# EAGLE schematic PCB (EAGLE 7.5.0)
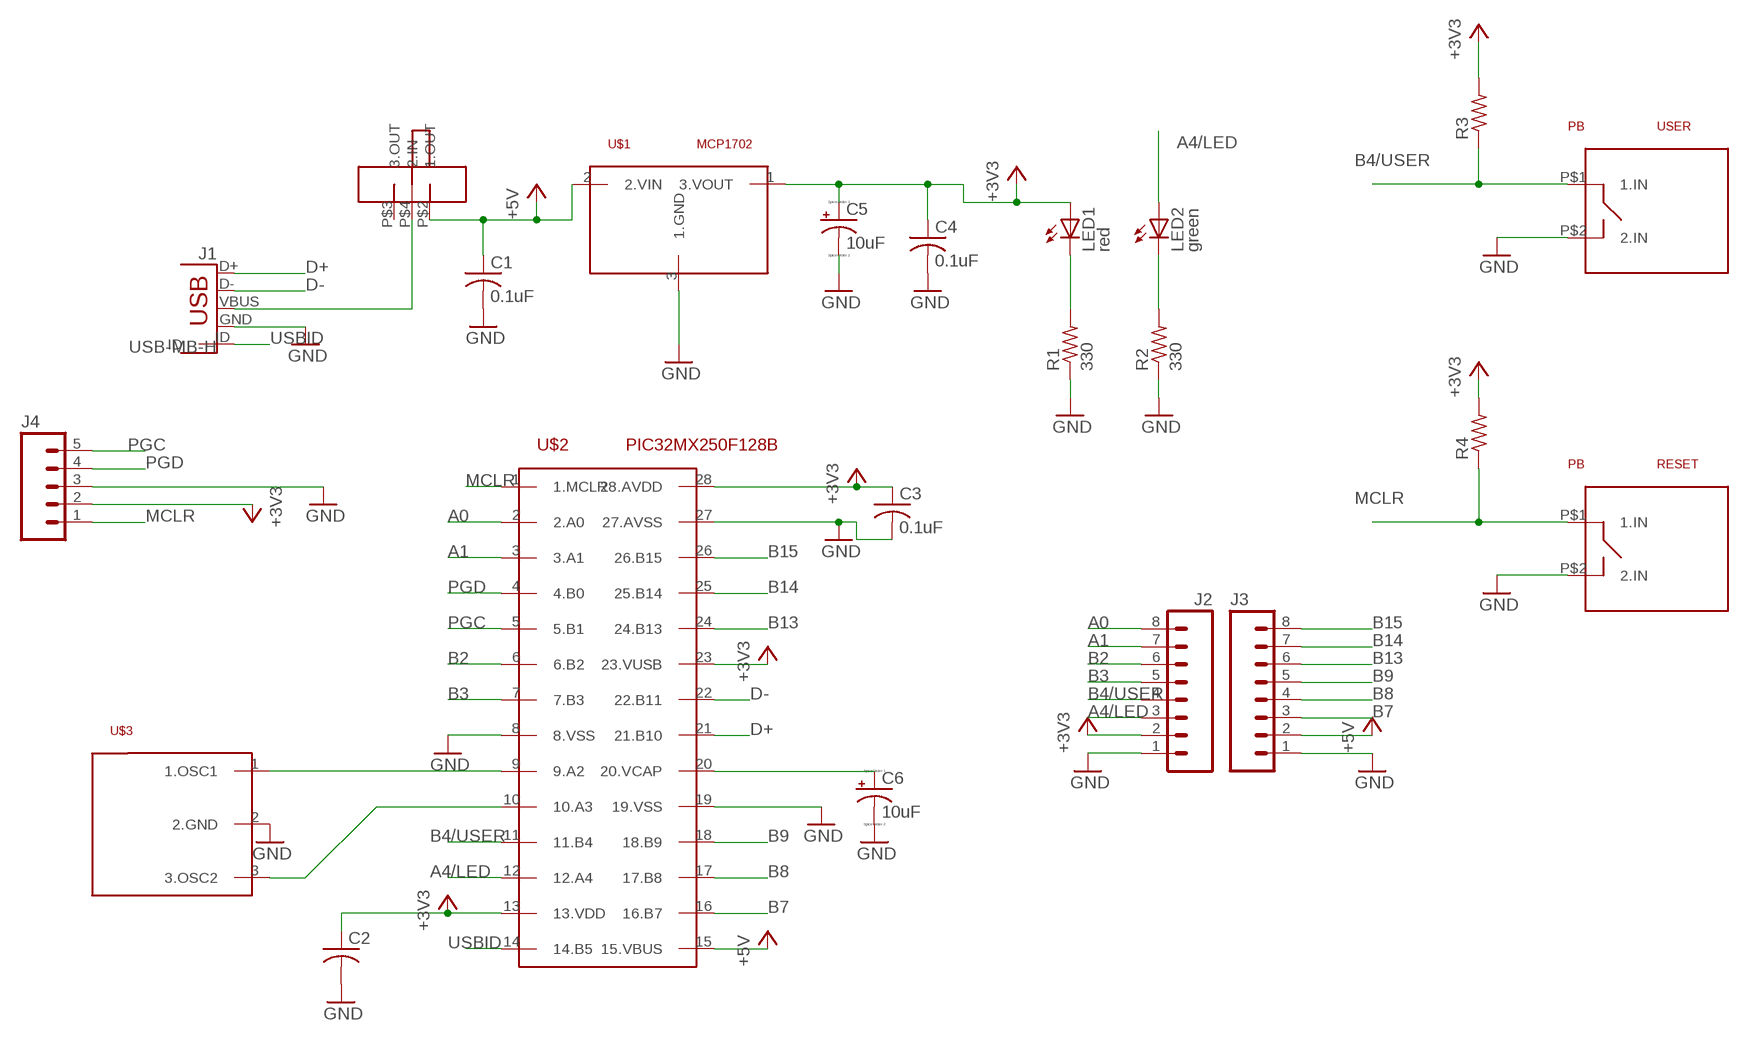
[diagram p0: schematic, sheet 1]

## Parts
C1  0.1uF  C-US025-025X050  [C025-025X050]
C2  C-US025-025X050  [C025-025X050]
C3  0.1uF  C-US025-025X050  [C025-025X050]
C4  0.1uF  C-US025-025X050  [C025-025X050]
C5  10uF  CPOL-USB45181A  [B45181A]
C6  10uF  CPOL-USB45181A  [B45181A]
J1  USB-MB-H  [USB-MB-H]
J2  M08  [1X08_ROUND]
J3  M08  [1X08_ROUND]
J4  M05PTH  [1X05]
LED1  red  LED3MM  [LED3MM]
LED2  green  LED3MM  [LED3MM]
R1  330  R-US_0207/10  [0207/10]
R2  330  R-US_0207/10  [0207/10]
R3  R-US_0207/10  [0207/10]
R4  R-US_0207/10  [0207/10]
RESET  PB  [PUSHBUTTON]
U$1  MCP1702  [TO92]
U$2  PIC32MX250F128B  [DIL28-3]
U$3  CRES  [1X03]
U$4  SLIDE  [SLIDE]
USER  PB  [PUSHBUTTON]

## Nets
+3V3: C2.1 C3.1 C4.1 C5.+ J2.2 J4.2 LED1.A R3.2 R4.2 U$1.1(3.VOUT) U$2.13(13.VDD) U$2.23(23.VUSB) U$2.28(28.AVDD)
+5V: C1.1 J3.2 U$1.2(2.VIN) U$2.15(15.VBUS) U$4.P$2(1.OUT)
A0: J2.8 U$2.2(2.A0)
A1: J2.7 U$2.3(3.A1)
A4/LED: J2.3 LED2.A U$2.12(12.A4)
B2: J2.6 U$2.6(6.B2)
B3: J2.5 U$2.7(7.B3)
B4/USER: J2.4 R3.1 U$2.11(11.B4) USER.P$1(1.IN)
B7: J3.3 U$2.16(16.B7)
B8: J3.4 U$2.17(17.B8)
B9: J3.5 U$2.18(18.B9)
B13: J3.6 U$2.24(24.B13)
B14: J3.7 U$2.25(25.B14)
B15: J3.8 U$2.26(26.B15)
D+: U$2.21(21.B10)
D-: J1.D-
GND: C1.2 C2.2 C3.2 C4.2 C5.- C6.- J1.GND J2.1 J3.1 J4.3 R1.1 R2.1 RESET.P$2(2.IN) U$1.3(1.GND) U$2.8(8.VSS) U$2.19(19.VSS) U$2.27(27.AVSS) U$3.2(2.GND) USER.P$2(2.IN)
MCLR: J4.1 R4.1 RESET.P$1(1.IN) U$2.1(1.MCLR)
N$1: J1.VBUS U$4.P$4(2.IN)
N$2: J1.D+
N$3: U$2.22(22.B11)
N$4: J1.ID
N$5: LED2.K(C) R2.2
N$8: LED1.K(C) R1.2
N$29: C6.+ U$2.20(20.VCAP)
N$36: U$2.10(10.A3) U$3.3(3.OSC2)
N$37: U$2.9(9.A2) U$3.1(1.OSC1)
PGC: J4.5 U$2.5(5.B1)
PGD: J4.4 U$2.4(4.B0)
USBID: U$2.14(14.B5)
Unconnected: U$4.P$3(3.OUT)

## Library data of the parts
C1-C4 = ME 433 PCB lib:C-US: CAPACITOR, American symbol
C5 C6 = ME 433 PCB lib:CPOL-US: POLARIZED CAPACITOR, American symbol
J1 = ME 433 PCB lib:USB: USB Connectors USB-B-PTH is fully proven SKU : PRT-00139/CONN-08278 USB-miniB is fully proven SKU : PRT-00587 USB-A-PCB is untested. USB-A-H is throughly reviewed, but untested. Spark Fun Electronics SKU : PRT-00437 USB-B-SMT is throughly reviewed, but untested. Needs silkscreen touching up.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
J2 J3 = ME 433 PCB lib:M08: Header 8 Standard 8-pin 0.1" header. Use with straight break away headers (SKU : PRT-00116), right angle break away headers (PRT-00553), swiss pins (PRT-00743), machine pins (PRT-00117), and female headers (PRT-00115).; PROD_ID: CONN-08437
J4 = ME 433 PCB lib:M05: Header 5 Standard 5-pin 0.1" header. Use with straight break away headers (SKU : PRT-00116), right angle break away headers (PRT-00553), swiss pins (PRT-00743), machine pins (PRT-00117), and female headers (PRT-00115). Molex polarized connector foot print use with SKU : PRT-08230 with associated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
LED1 LED2 = ME 433 PCB lib:LED: LED
R1-R4 = ME 433 PCB lib:R-US_: RESISTOR, American symbol
RESET USER = ME 433 PCB lib:PB
U$1 = ME 433 PCB lib:MCP1702
U$2 = ME 433 PCB lib:PIC32MX250F128B
U$3 = ME 433 PCB lib:CRES
U$4 = ME 433 PCB lib:SLIDE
